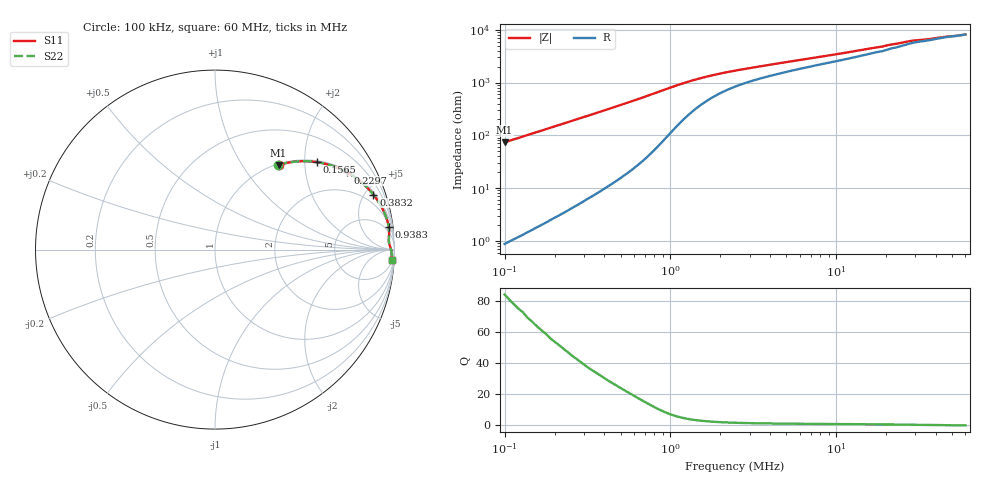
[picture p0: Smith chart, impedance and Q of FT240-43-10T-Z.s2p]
! ListType=Log
!!FT240-43 10T Z
# MHZ S RI R 50
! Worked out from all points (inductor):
!   101 points, 100 kHz to 60 MHz, reference 50 ohm
!   read as one part in series: L = 117 uH near 100 kHz
!   highest Q = 84.4 at 100 kHz (marker M1), where L = 117 uH
!   S11 on the Smith chart (normalised r, x): 100 kHz: 1.02, +1.47; 156.5 kHz: 1.04, +2.31; 229.7 kHz: 1.07, +3.39; 383.2 kHz: 1.19, +5.70; 938.3 kHz: 3, +15; 60 MHz: 8, -32
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0.1  0.3538 0.472  0.6465 -0.4725  0.6466 -0.4725  0.3537 0.472
0.1291594  0.4757 0.4923  0.5245 -0.4929  0.5246 -0.4929  0.4756 0.4924
0.1564842  0.5698 0.4871  0.4304 -0.4877  0.4305 -0.4878  0.5697 0.4871
0.1895899  0.6588 0.4649  0.3414 -0.4657  0.3415 -0.4657  0.6587 0.465
0.2296993  0.7375 0.4296  0.2626 -0.4302  0.2626 -0.4303  0.7374 0.4296
0.2966783  0.8218 0.3699  0.1781 -0.3705  0.1781 -0.3706  0.8218 0.37
0.3831879  0.8826 0.306  0.1173 -0.3067  0.1173 -0.3068  0.8826 0.3061
0.4642547  0.9149 0.26  0.0849 -0.2607  0.0849 -0.2608  0.9149 0.2601
0.5624719  0.9381 0.2175  0.0617 -0.2183  0.0617 -0.2183  0.9382 0.2176
0.8801799  0.9662 0.135  0.0336 -0.136  0.0336 -0.1361  0.9662 0.135
0.9383242  0.9678 0.1254  0.032 -0.1264  0.032 -0.1264  0.9678 0.1254
1.211934  0.9699 0.0931  0.0299 -0.0944  0.0299 -0.0944  0.9699 0.0931
1.565327  0.9691 0.0706  0.0306 -0.0722  0.0306 -0.0722  0.9692 0.0705
2.021767  0.9686 0.055  0.0312 -0.057  0.0312 -0.057  0.9687 0.0549
2.611302  0.9689 0.0437  0.0309 -0.0463  0.0309 -0.0463  0.9688 0.0437
7.267103  0.9759 0.0161  0.0237 -0.0232  0.0237 -0.0232  0.9758 0.0161
18.97073  0.9825 -0.00696  0.0166 -0.0118  0.0166 -0.0118  0.9825 -0.00696
21.55992  0.9827 -0.0103  0.0156 -0.0101  0.0156 -0.0102  0.9828 -0.0103
27.84666  0.9835 -0.0187  0.0143 -0.00727  0.0143 -0.00729  0.9835 -0.0187
35.96658  0.9846 -0.0291  0.014 -0.00502  0.014 -0.00505  0.9846 -0.0292
43.57563  0.9844 -0.0386  0.0132 -0.00346  0.0132 -0.00348  0.9845 -0.0387
60  0.9837 -0.058  0.012 -0.000767  0.0121 -0.000789  0.984 -0.0582
